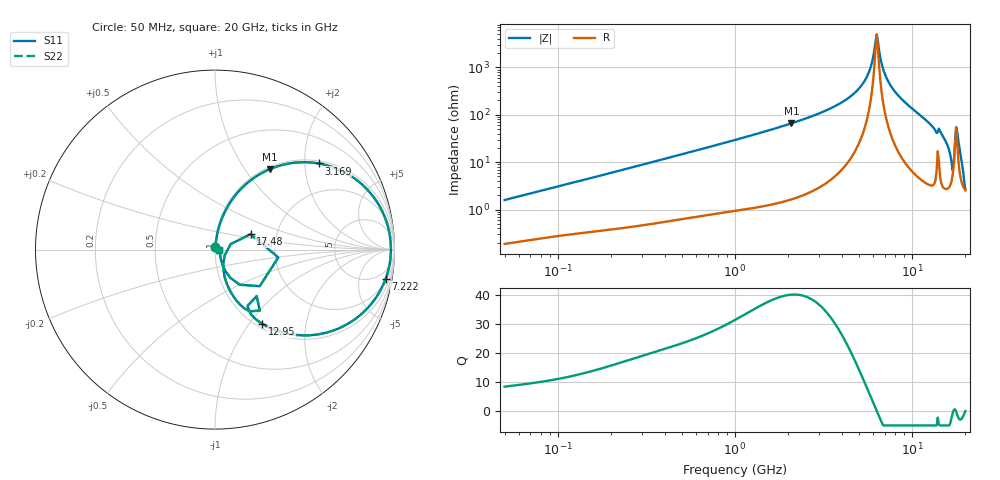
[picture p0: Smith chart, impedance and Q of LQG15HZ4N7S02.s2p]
!Murata Part Number: LQG15HZ4N7S02
!These Parameters are Measured in Series Mode Connection
!  o--[Z]--o
!Port1  Port2
!  o-------o
!Freq. Start=50[MHz] Stop=20[GHz], 401[Steps]
# Hz S RI R 50
!Freq.(Hz) S11(Real) S11(Imag) S21(Real) S21(Imag) S12(Real) S12(Imag) S22(Real) S22(Imag)
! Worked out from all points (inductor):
!   401 points, 50 MHz to 20 GHz, reference 50 ohm
!   read as one part in series: L = 4.98 nH near 51.52 MHz
!   highest Q = 40.1 at 2.083 GHz (marker M1), where L = 5.03 nH
!   self-resonance near 6.312 GHz
!   S11 on the Smith chart (normalised r, x): 50 MHz: 1.00, +0.03; 3.169 GHz: 1.07, +2.34; 7.222 GHz: 2, -11; 12.95 GHz: 1.06, -1.16; 17.48 GHz: 1.47, +0.26; 20 GHz: 1.05, -0.00
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5e7  0.00214 0.0158  0.9979 -0.0158  0.9979 -0.0158  0.00214 0.0158
1.364002e8  0.00487 0.0408  0.9951 -0.0408  0.9951 -0.0408  0.00487 0.0408
3.721004e8  0.0169 0.107  0.9831 -0.107  0.9831 -0.107  0.0169 0.107
1e9  0.0867 0.2659  0.9133 -0.2659  0.9133 -0.2659  0.0867 0.2659
2.083303e9  0.3072 0.449  0.6928 -0.449  0.6928 -0.449  0.3072 0.449
2.728004e9  0.4678 0.4861  0.5322 -0.4861  0.5322 -0.4861  0.4678 0.4861
3.168813e9  0.5768 0.48  0.4232 -0.48  0.4232 -0.48  0.5768 0.48
4.212059e9  0.7982 0.3809  0.2018 -0.3809  0.2018 -0.3809  0.7982 0.3809
5.117541e9  0.9234 0.2303  0.0766 -0.2303  0.0766 -0.2303  0.9234 0.2303
5.683258e9  0.9652 0.1224  0.0348 -0.1224  0.0348 -0.1224  0.9652 0.1224
6.311513e9  0.9802 0.000825  0.0198 -0.000825  0.0198 -0.000825  0.9802 0.000825
6.802353e9  0.971 -0.0903  0.029 0.0903  0.029 0.0903  0.971 -0.0903
7.222371e9  0.9506 -0.163  0.0494 0.163  0.0494 0.163  0.9506 -0.163
7.442007e9  0.9358 -0.1987  0.0642 0.1987  0.0642 0.1987  0.9358 -0.1987
1.004137e10  0.6346 -0.4586  0.3654 0.4586  0.3654 0.4586  0.6346 -0.4586
1.295331e10  0.2628 -0.4132  0.7372 0.4132  0.7372 0.4132  0.2628 -0.4132
1.504638e10  0.1202 -0.2848  0.8798 0.2848  0.8798 0.2848  0.1202 -0.2848
1.670968e10  0.0459 -0.084  0.9541 0.084  0.9541 0.084  0.0459 -0.084
1.747767e10  0.198 0.0858  0.802 -0.0858  0.802 -0.0858  0.198 0.0858
1.800918e10  0.2491 -0.204  0.7509 0.204  0.7509 0.204  0.2491 -0.204
1.828096e10  0.1379 -0.1959  0.8621 0.1959  0.8621 0.1959  0.1379 -0.1959
2e10  0.0251 -0.000612  0.9749 0.000612  0.9749 0.000612  0.0251 -0.000612
